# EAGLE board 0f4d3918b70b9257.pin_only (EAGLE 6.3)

Size 25.4 x 14.1 mm. Coordinates in mm from the lower left corner, seen from the top.
Outline: 0,12.19 0,1.91 arc90 1.91,0 23.5,0 arc90 25.4,1.91 25.4,12.19 arc90 23.5,14.1 1.91,14.1 arc90 0,12.19
Copper layers (1*16): Top 0.035mm / dielectric 1.5mm / Bottom 0.035mm
Design rules "adafruit *": minimum track width 8mil, minimum drill 15.5mil, track to track 7mil, track to pad 7mil, pad to pad 7mil, via to via 7mil, smd to smd 7mil, copper to edge 10mil, drill to drill 8mil, minimum pad ring 10mil, minimum via ring 8mil, stop-mask expansion 4mil, vias tented up to drill 20mil, thermal gap 10mil

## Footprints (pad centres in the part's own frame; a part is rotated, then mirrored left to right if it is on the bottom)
C0805K = smd 1.1 x 1.4: 1 -1,0; 2 1,0
0805 = smd 1.3 x 1.5: 1 -0.95,0; 2 0.95,0
1X05_ROUND_76 = drill 1 pad 1.93: 1 -5.08,0; 2 -2.54,0; 3 0,0; 4 2.54,0; 5 5.08,0
9.7ELECTRET = drill 0.6 pad 1.778: + 1.3,2; - -1.3,2
R0805 = smd 1.1 x 1.4: 1 -1,0; 2 1,0
TDFN14_3X3MM = smd 0.7 x 0.2: P$1 -1.475,1.2; P$2 -1.475,0.8; P$3 -1.475,0.4; P$4 -1.475,0; P$5 -1.475,-0.4; P$6 -1.475,-0.8; P$7 -1.475,-1.2; P$8 1.475,-1.2; P$9 1.475,-0.8; P$10 1.475,-0.4; P$11 1.475,0; P$12 1.475,0.4; P$13 1.475,0.8; P$14 1.475,1.2 | smd 1.27 x 2.35: P$THERMAL 0,0
FIDUCIAL_1MM = smd 1 x 1: 1 0,0
MOUNTINGHOLE_2.0_PLATED = drill 2.2 pad 3: P$1 0,0

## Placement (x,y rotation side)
C1  2.2uF  [C0805K]  7.49,10.54 90 top
C2  0.1uF  [C0805K]  10.92,10.54 90 top
C5  2.2uF  [C0805K]  7.49,5.97 270 top
C8  0.47uF  [C0805K]  17.02,6.1 0 top
C9  0.1uF  [C0805K]  16.26,2.03 0 top
FB1  FERRITE  [0805]  5.21,6.48 90 top
FB2  FERRITE  [0805]  5.21,10.54 90 top
J2  [1X05_ROUND_76]  1.4,6.86 270 top
Q1  CMA-4544PF-W  [9.7ELECTRET]  18.16,7.11 90 bottom
R1  150k  [R0805]  17.02,10.29 0 top
R2  100k  [R0805]  13.08,10.54 270 top
R3  2.2K  [R0805]  17.02,8.26 180 top
U$1  MAX9814TDFN14  [TDFN14_3X3MM]  11.81,6.35 0 top
U$2  FIDUCIAL  [FIDUCIAL_1MM]  5.46,1.91 0 top
U$3  FIDUCIAL  [FIDUCIAL_1MM]  15.49,12.45 0 top
U$4  MOUNTINGHOLE2.0  [MOUNTINGHOLE_2.0_PLATED]  23.37,12.06 0 top
U$5  MOUNTINGHOLE2.0  [MOUNTINGHOLE_2.0_PLATED]  23.37,2.03 0 top
U$6  [ADAFRUIT_3.5MM]  24.77,5.21 90 top

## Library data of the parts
C1 C2 C5 C8 C9 Q1 R1-R3 U$1-U$3 = adafruit
FB1 FB2 J2 U$4-U$6 = microbuilder

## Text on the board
tPlace: AGC Mic Amp | GND | V+ | G | Out | MAX9814 | AR | adafruit!
bPlace: DC Offset: 1.25V | Output 2Vpp max | Gain float->60dB | G=Vdd -> 40dB | G=Gnd -> 50dB | GND | Vdd | Gain | Out | AR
